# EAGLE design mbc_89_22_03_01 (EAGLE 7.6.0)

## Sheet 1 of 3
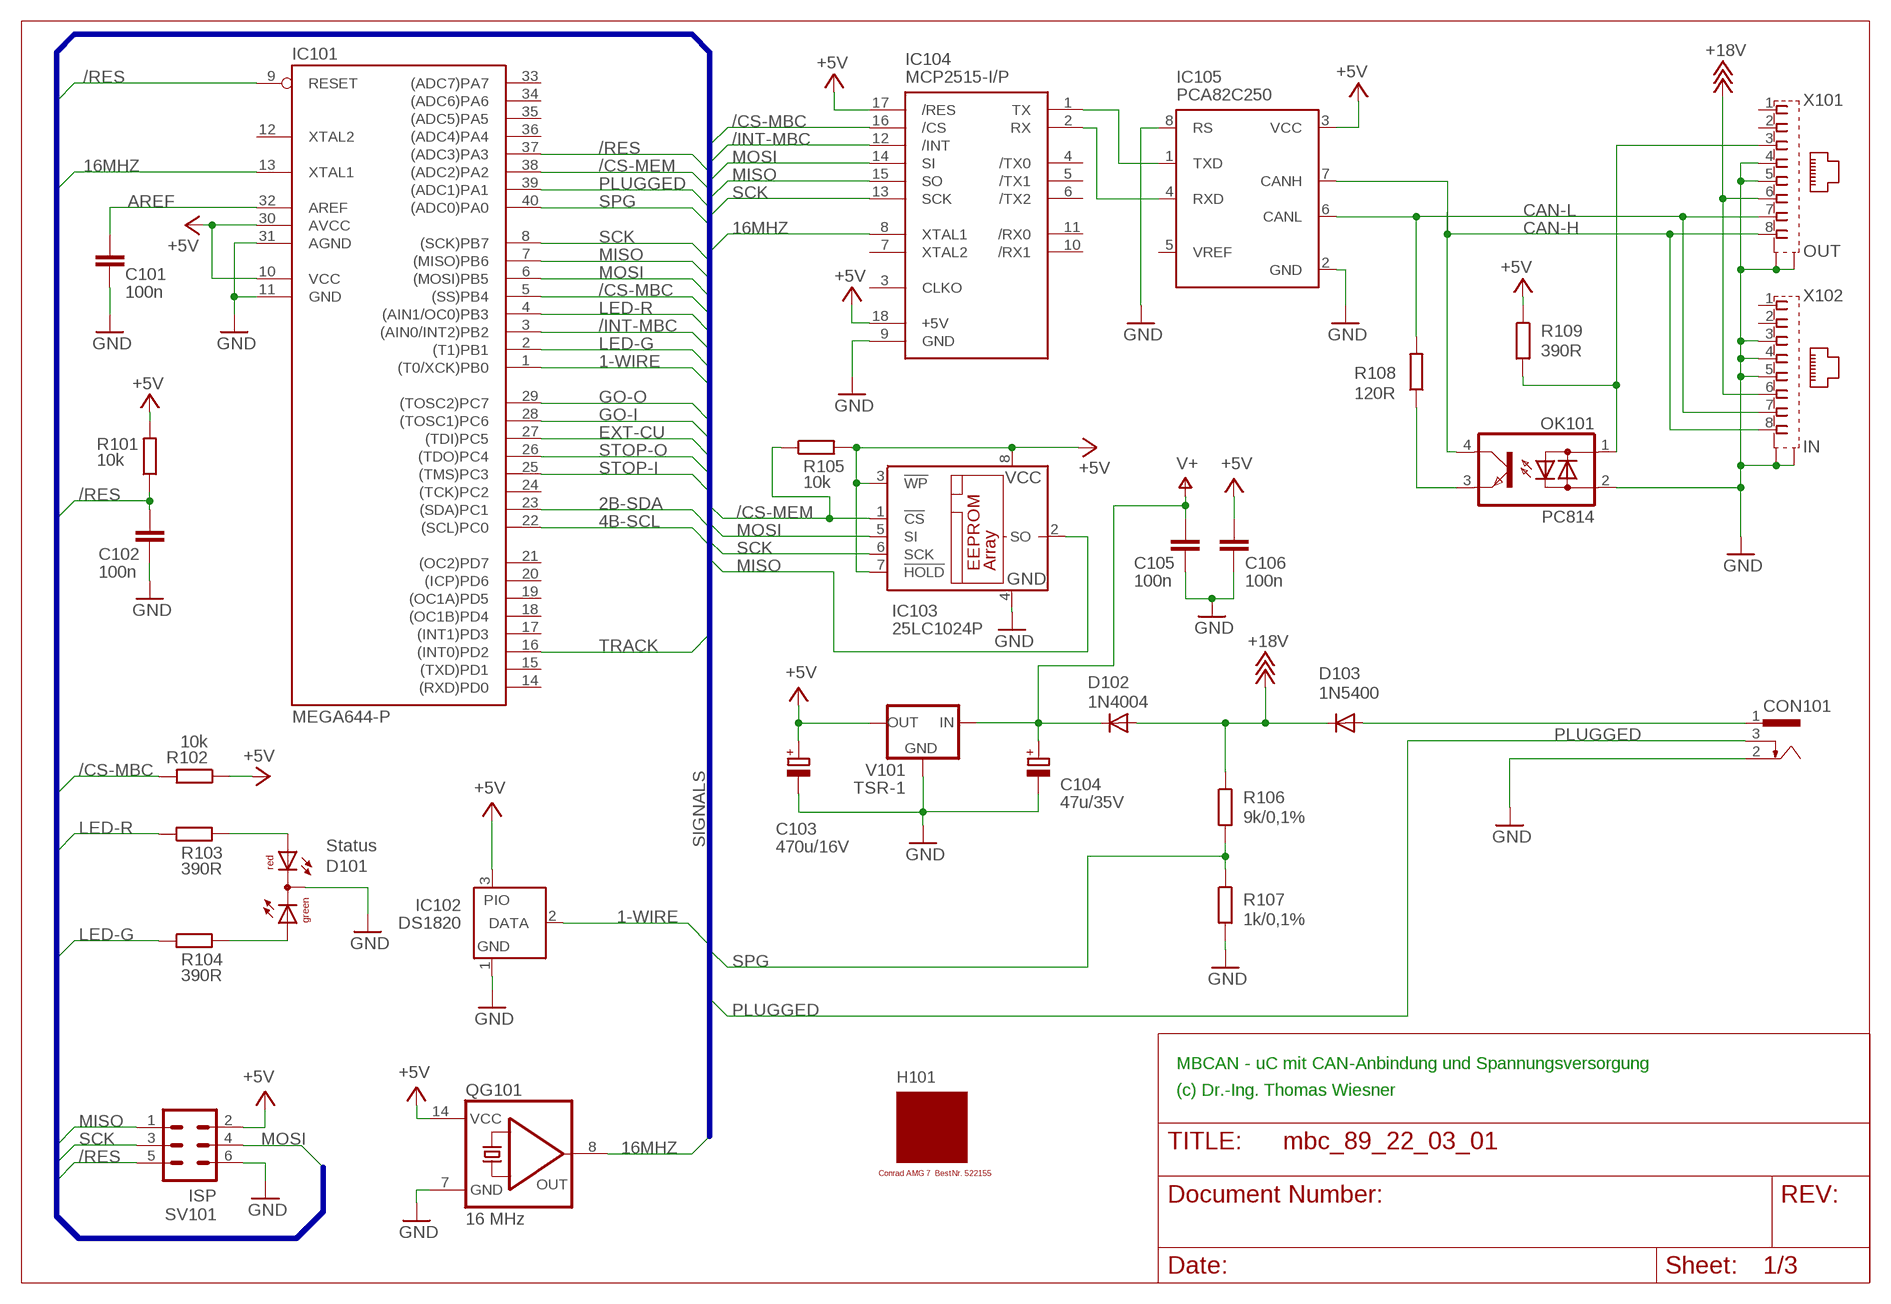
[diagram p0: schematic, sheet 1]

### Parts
C101  100n  C-EU025-025X050  [C025-025X050]
C102  100n  C-EU025-025X050  [C025-025X050]
C103  470u/16V  CPOL-EUE3.5-8  [E3,5-8]
C104  47u/35V  CPOL-EUE2.5-7  [E2,5-7]
C105  100n  C-EU025-025X050  [C025-025X050]
C106  100n  C-EU025-025X050  [C025-025X050]
CON101  POWER-JACK  [POWER-JACK]
D101  Status  DUOLED5MM  [DUOLED5MM]
D102  1N4004  [DO41-10]
D103  1N5400  [DO201-15]
H101  MODULGEHÄUSE-AMG-7  [MODULGEHÄUSE-1]
IC101  MEGA644-P  MEGA323-P  [DIL40]
IC102  DS1820  DS2405  [TO92-]
IC103  25LC1024P  25LC040P  [DIL8]
IC104  MCP2515-I/P  MCP2510-I/P  [DIL18]
IC105  PCA82C250  [DIL08]
OK101  PC814  [DIL04]
QG101  16 MHz  QG5860  [DIL14S]
R101  10k  R-EU_0207/10  [0207/10]
R102  10k  R-EU_0207/10  [0207/10]
R103  390R  R-EU_0207/10  [0207/10]
R104  390R  R-EU_0207/10  [0207/10]
R105  10k  R-EU_0207/10  [0207/10]
R106  9k/0,1%  R-EU_0207/10  [0207/10]
R107  1k/0,1%  R-EU_0207/10  [0207/10]
R108  120R  R-EU_0207/10  [0207/10]
R109  390R  R-EU_0207/10  [0207/10]
SV101  ISP  ML6  [ML6]
V101  TSR-1  [TRACO-TSR-1]
X101  OUT  0446200002  [0446200002]
X102  IN  0446200002  [0446200002]

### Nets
1-WIRE: IC101.1((T0/XCK)PB0) IC102.2(DATA)
2B-SDA: IC101.23((SDA)PC1) ; also sheet 2
4B-SCL: IC101.22((SCL)PC0) ; also sheet 2
16MHZ: IC101.13(XTAL1) IC104.8(XTAL1) QG101.8(OUT)
+5V: C103.+ C106.1 IC101.10(VCC) IC101.30(AVCC) IC102.3(PIO) IC103.3(!WP) IC103.7(!HOLD) IC103.8(VCC) IC104.17(/RES) IC104.18(+5V) IC105.3(VCC) QG101.14(VCC) R101.2 R102.1 R105.2 R109.1 SV101.2 V101.OUT ; also sheet 2
+18V: D102.A D103.C R106.1 X101.6 X102.6
/CS-MBC: IC101.5((SS)PB4) IC104.16(/CS) R102.2
/CS-MEM: IC101.38((ADC2)PA2) IC103.1(!CS) R105.1
/INT-MBC: IC101.3((AIN0/INT2)PB2) IC104.12(/INT)
/RES: C102.1 IC101.9(RESET) IC101.37((ADC3)PA3) R101.1 SV101.5
AREF: C101.1 IC101.32(AREF)
CAN-H: IC105.7(CANH) OK101.4(C) X101.8 X102.8
CAN-L: IC105.6(CANL) R108.2 X101.7 X102.7
EXT-CU: IC101.27((TDI)PC5) ; also sheet 2
GND: C101.2 C102.2 C103.- C104.- C105.2 C106.2 CON101.2 D101.K(C) IC101.11(GND) IC101.31(AGND) IC102.1(GND) IC103.4(GND) IC104.9(GND) IC105.2(GND) IC105.8(RS) OK101.2(AC2) QG101.7(GND) R107.2 SV101.6 V101.GND X101.4 X101.5 X101.S@1(S1) X101.S@2(S2) X102.3 X102.4 X102.5 X102.S@1(S1) X102.S@2(S2) ; also sheet 2
GO-I: IC101.28((TOSC1)PC6) ; also sheet 2
GO-O: IC101.29((TOSC2)PC7) ; also sheet 2
LED-G: IC101.2((T1)PB1) R104.1
LED-R: IC101.4((AIN1/OC0)PB3) R103.1
MISO: IC101.7((MISO)PB6) IC103.2(SO) IC104.15(SO) SV101.1
MOSI: IC101.6((MOSI)PB5) IC103.5(SI) IC104.14(SI) SV101.4
N$1: IC104.1(TX) IC105.1(TXD)
N$2: IC104.2(RX) IC105.4(RXD)
N$5: OK101.3(E) R108.1
N$9: D101.AR R103.2
N$11: OK101.1(AC1) R109.2 X101.3
N$13: D101.AG R104.2
PLUGGED: CON101.3 IC101.39((ADC1)PA1)
SCK: IC101.8((SCK)PB7) IC103.6(SCK) IC104.13(SCK) SV101.3
SPG: IC101.40((ADC0)PA0) R106.2 R107.1
STOP-I: IC101.25((TMS)PC3) ; also sheet 2
STOP-O: IC101.26((TDO)PC4) ; also sheet 2
TRACK: IC101.16((INT0)PD2) ; also sheet 2
V+: C104.+ C105.1 D102.C V101.IN ; also sheet 2
V-NETZTEIL: CON101.1 D103.A
Unconnected: IC101.12(XTAL2) IC101.14((RXD)PD0) IC101.15((TXD)PD1) IC101.17((INT1)PD3) IC101.18((OC1B)PD4) IC101.19((OC1A)PD5) IC101.20((ICP)PD6) IC101.21((OC2)PD7) IC101.24((TCK)PC2) IC101.33((ADC7)PA7) IC101.34((ADC6)PA6) IC101.35((ADC5)PA5) IC101.36((ADC4)PA4) IC104.3(CLKO) IC104.4(/TX0) IC104.5(/TX1) IC104.6(/TX2) IC104.7(XTAL2) IC104.10(/RX1) IC104.11(/RX0) IC105.5(VREF) X101.1 X101.2 X102.1 X102.2

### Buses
SIGNALS

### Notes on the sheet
- MBCAN - uC mit CAN-Anbindung und Spannungsversorgung
- (c) Dr.-Ing. Thomas Wiesner

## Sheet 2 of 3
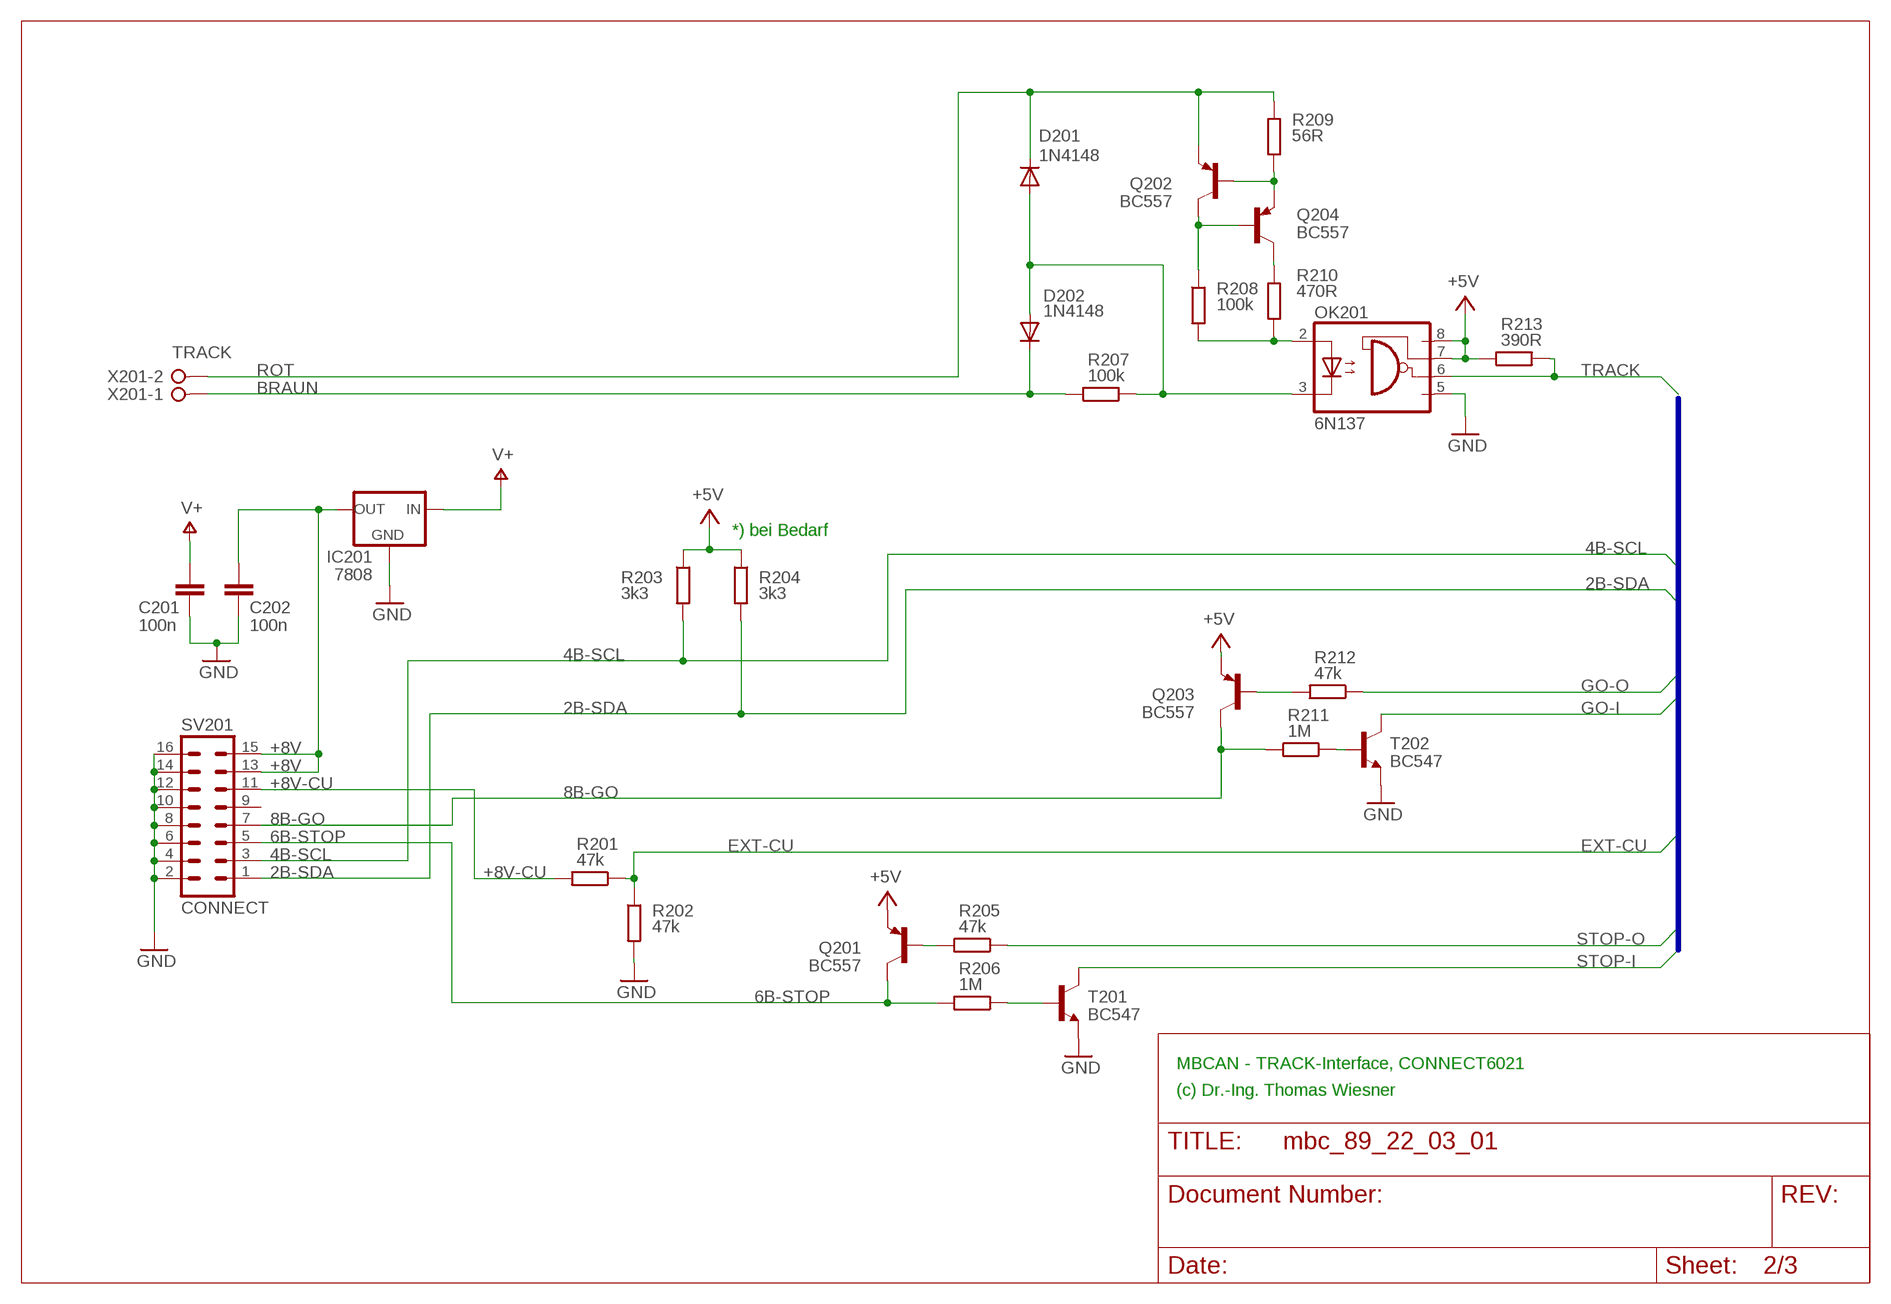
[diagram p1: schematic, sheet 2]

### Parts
C201  100n  C-EU025-025X050  [C025-025X050]
C202  100n  C-EU025-025X050  [C025-025X050]
D201  1N4148  1N4148DO35-10  [DO35-10]
D202  1N4148  1N4148DO35-10  [DO35-10]
IC201  7808  78XXL  [78XXL]
OK201  6N137  [DIL08]
Q201  BC557  [TO92]
Q202  BC557  [TO92]
Q203  BC557  [TO92]
Q204  BC557  [TO92]
R201  47k  R-EU_0207/10  [0207/10]
R202  47k  R-EU_0207/10  [0207/10]
R203  3k3  R-EU_0207/10  [0207/10]
R204  3k3  R-EU_0207/10  [0207/10]
R205  47k  R-EU_0207/10  [0207/10]
R206  1M  R-EU_0207/10  [0207/10]
R207  100k  R-EU_0207/10  [0207/10]
R208  100k  R-EU_0207/10  [0207/10]
R209  56R  R-EU_0207/10  [0207/10]
R210  470R  R-EU_0207/10  [0207/10]
R211  1M  R-EU_0207/10  [0207/10]
R212  47k  R-EU_0207/10  [0207/10]
R213  390R  R-EU_0207/10  [0207/10]
SV201  CONNECT  ML16  [ML16]
T201  BC547  [TO92]
T202  BC547  [TO92]
X201  TRACK  W237-02P  [W237-132]

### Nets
2B-SDA: R204.2 SV201.1 ; also sheet 1
4B-SCL: R203.2 SV201.3 ; also sheet 1
6B-STOP: Q201.3(C) R206.2 SV201.5
8B-GO: Q203.3(C) R211.2 SV201.7
+5V: OK201.7(VE) OK201.8(VCC) Q201.1(E) Q203.1(E) R203.1 R204.1 R213.1 ; also sheet 1
+8V: C202.1 IC201.OUT SV201.13 SV201.15
+8V-CU: R201.2 SV201.11
BRAUN: D202.C R207.2 X201.1
EXT-CU: R201.1 R202.1 ; also sheet 1
GND: C201.2 C202.2 IC201.GND OK201.5(GND) R202.2 SV201.2 SV201.4 SV201.6 SV201.8 SV201.10 SV201.12 SV201.14 SV201.16 T201.1(E) T202.1(E) ; also sheet 1
GO-I: T202.3(C) ; also sheet 1
GO-O: R212.1 ; also sheet 1
N$3: R206.1 T201.2(B)
N$4: Q201.2(B) R205.2
N$7: R211.1 T202.2(B)
N$12: Q203.2(B) R212.2
N$43: D201.A D202.A OK201.3(C) R207.1
N$53: Q202.2(B) Q204.1(E) R209.2
N$54: Q202.3(C) Q204.2(B) R208.1
N$56: Q204.3(C) R210.1
N$57: OK201.2(A) R208.2 R210.2
ROT: D201.C Q202.1(E) R209.1 X201.2
STOP-I: T201.3(C) ; also sheet 1
STOP-O: R205.1 ; also sheet 1
TRACK: OK201.6(VO) R213.2 ; also sheet 1
V+: C201.1 IC201.IN ; also sheet 1
Unconnected: SV201.9

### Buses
B$1
SIGNALS

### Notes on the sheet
- *) bei Bedarf
- MBCAN - TRACK-Interface, CONNECT6021
- (c) Dr.-Ing. Thomas Wiesner

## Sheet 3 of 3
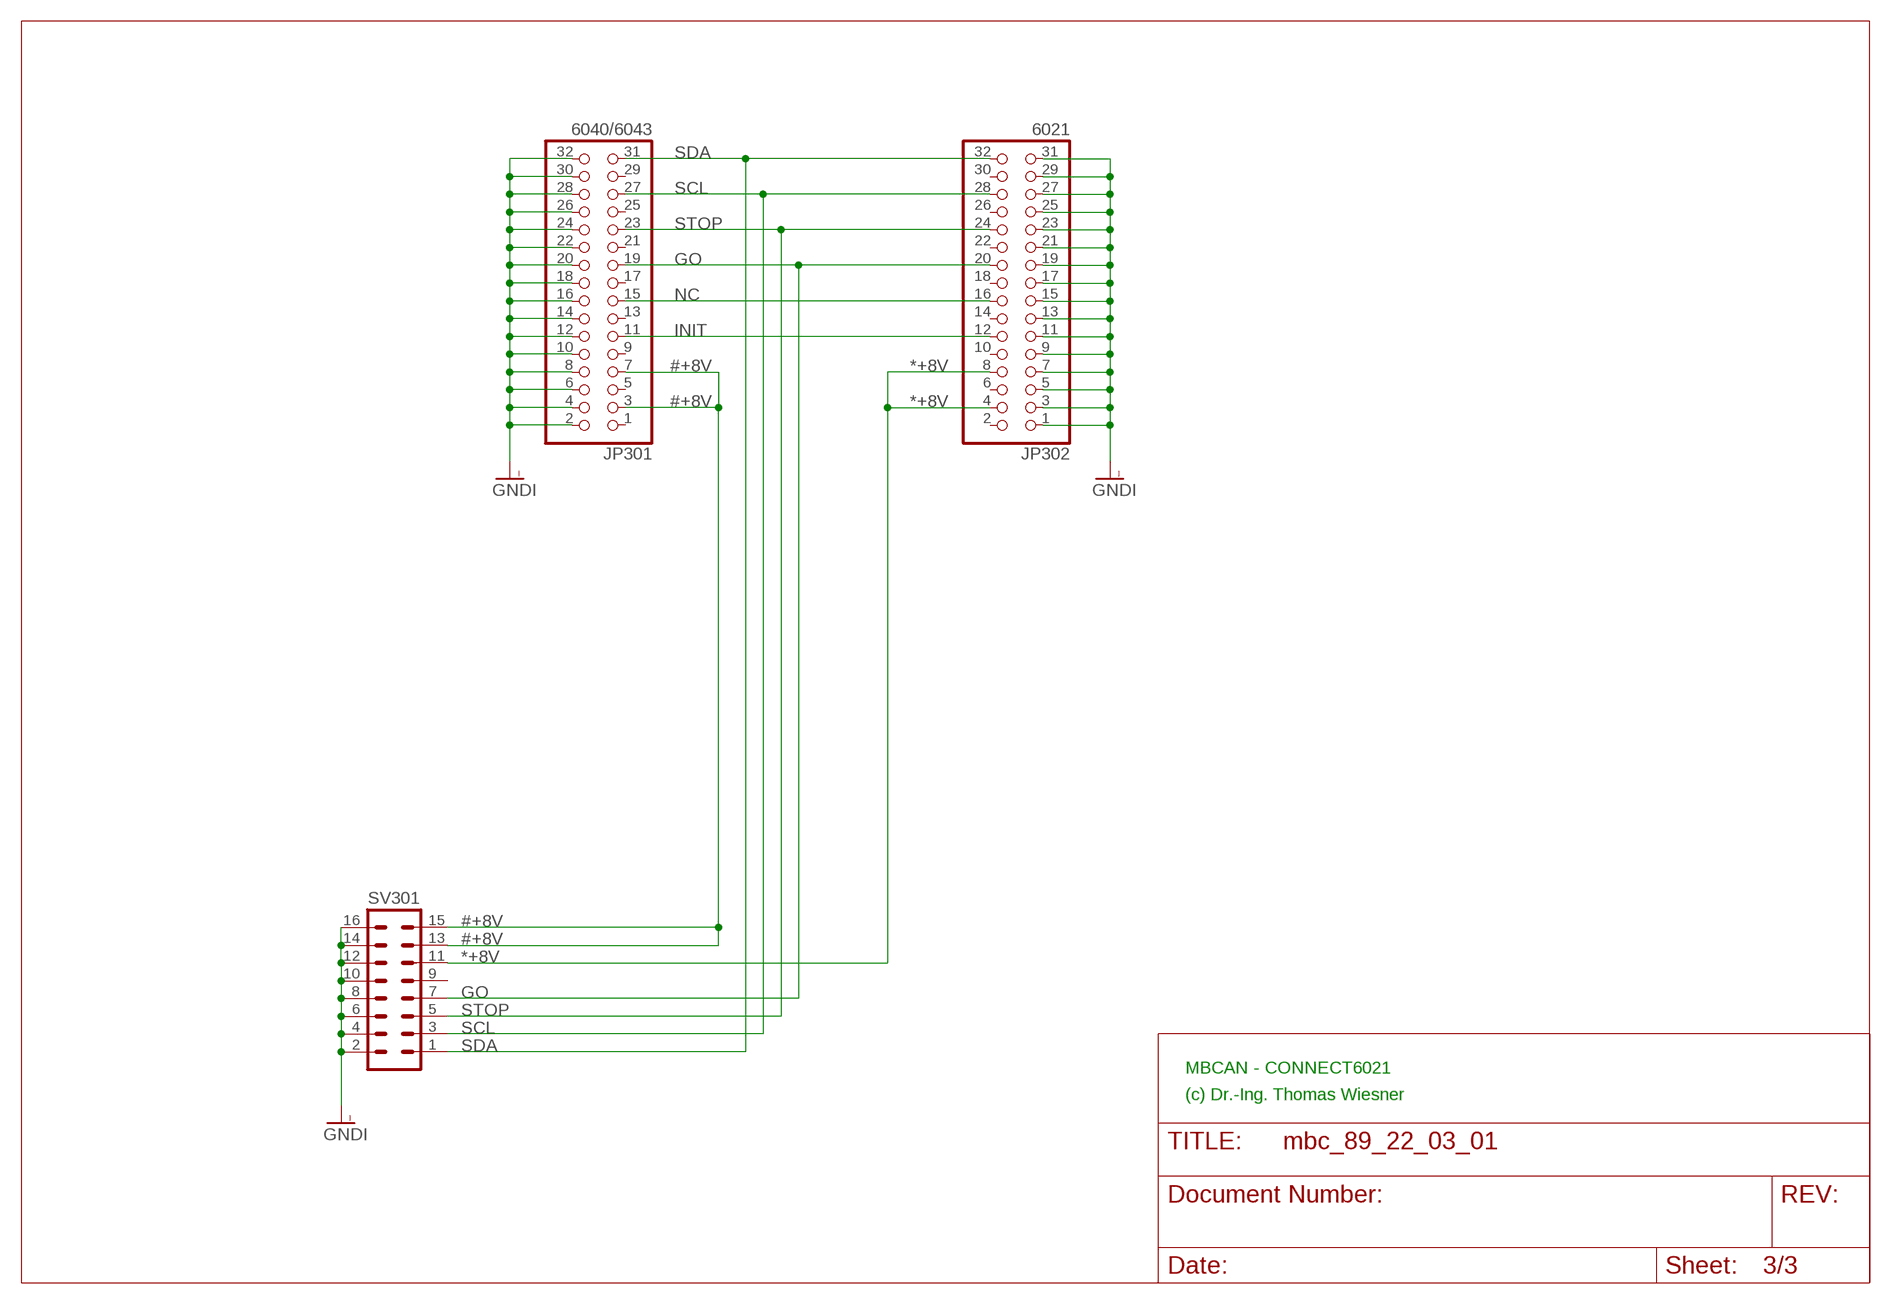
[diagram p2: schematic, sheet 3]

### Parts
JP301  6040/6043  PINHD-2X16  [2X16]
JP302  6021  PINHD-2X16  [2X16]
SV301  ML16  [ML16]

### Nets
#+8V: JP301.3 JP301.7 SV301.13 SV301.15
*+8V: JP302.4 JP302.8 SV301.11
GNDI: JP301.2 JP301.4 JP301.6 JP301.8 JP301.10 JP301.12 JP301.14 JP301.16 JP301.18 JP301.20 JP301.22 JP301.24 JP301.26 JP301.28 JP301.30 JP301.32 JP302.1 JP302.3 JP302.5 JP302.7 JP302.9 JP302.11 JP302.13 JP302.15 JP302.17 JP302.19 JP302.21 JP302.23 JP302.25 JP302.27 JP302.29 JP302.31 SV301.2 SV301.4 SV301.6 SV301.8 SV301.10 SV301.12 SV301.14 SV301.16
GO: JP301.19 JP302.20 SV301.7
INIT: JP301.11 JP302.12
NC: JP301.15 JP302.16
SCL: JP301.27 JP302.28 SV301.3
SDA: JP301.31 JP302.32 SV301.1
STOP: JP301.23 JP302.24 SV301.5
Unconnected: JP301.1 JP301.5 JP301.9 JP301.13 JP301.17 JP301.21 JP301.25 JP301.29 JP302.2 JP302.6 JP302.10 JP302.14 JP302.18 JP302.22 JP302.26 JP302.30 SV301.9

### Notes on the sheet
- MBCAN - CONNECT6021
- (c) Dr.-Ing. Thomas Wiesner

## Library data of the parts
C101 C102 C105 C106 C201 C202 = rcl:C-EU: CAPACITOR, European symbol
C103 C104 = rcl:CPOL-EU: POLARIZED CAPACITOR, European symbol
CON101 = mbc:POWER-JACK
D101 = led:DUOLED5MM: DUO LED 2 colors, 5 mm, round
D102 = diode:1N4004: DIODE
D103 = diode:1N5400: DIODE
D201 D202 = diode:1N4148: DIODE
H101 = mbc:MODULGEHÄUSE-AMG-7: Gehäuse
IC101 = atmel:MEGA323-P: MICROCONTROLLER 32 Kbytes FLASH 2 Kbytes SRAM 1 Kbytes EEPROM USART 8-channel 10 bit ADC Source: avr.lbr; OC_FARNELL: unknown; OC_NEWARK: unknown
IC102 = maxim:DS2405: Addressable Switch DALLAS Semiconductor; MF: DALLAS SEMICONDUCTOR; MPN: DS2405; OC_FARNELL: 1188025; OC_NEWARK: 06F4645
IC103 = microchip:25*: Serial EEPROM 4K/ 8K , SPI bus; MF: MICROCHIP; MPN: 25LC040/P; OC_FARNELL: 9758100; OC_NEWARK: 96K4091
IC104 = mbc:MCP2510: BASIC-CAN 2.0a Controller Stand-alone CAN controller von Microchip
IC105 = micro-philips:PCA82C250: CAN CONTROLLER INTERFACE; OC_FARNELL: 3692358; OC_NEWARK: unknown
IC201 = v-reg:78XXL: VOLTAGE REGULATOR
JP301 JP302 = pinhead:PINHD-2X16: PIN HEADER
OK101 = optocoupler:PC814: SHARP OPTO COUPLER; OC_FARNELL: 9707662; OC_NEWARK: unknown
OK201 = optocoupler:6N137: MOTOROLA OPTO COUPLER; MPN: 6N137; OC_FARNELL: 1328376; OC_NEWARK: 52M1895
Q201-Q204 = transistor-pnp:BC557: PNP Transistor
QG101 = crystal:QG5860: CRYSTAL RESONATOR; OC_FARNELL: unknown; OC_NEWARK: unknown
R101-R109 R201-R213 = resistor:R-EU_: RESISTOR, European symbol
SV101 = con-ml:ML6: HARTING; OC_FARNELL: unknown; OC_NEWARK: unknown
SV201 SV301 = con-ml:ML16: HARTING; OC_FARNELL: unknown; OC_NEWARK: unknown
T201 T202 = transistor:BC547: NPN TRANSISTOR
V101 = mbc:TSR-1: Spannungsregler Hersteller: TRACO Typ: TSR-1 5V: TSR 1-2450 Spg: 5V Strom: 1A Reichelt TSR 1-2450
X101 X102 = mbc:0446200002: RJ-45 INVERTED MODULAR JACK ASSEMBLY WITH RJ-11 KEEPOUT FEATURE Source: Data sheet MOLEX 0446200002 BUCHSE, RJ45, GESCHIRMT Source: Farnell; MF: MOLEX; MPN: 0446200002; OC_FARNELL: 9251910
X201 = con-wago-508:W237-02P: WAGO SREW CLAMP; OC_FARNELL: unknown; OC_NEWARK: unknown

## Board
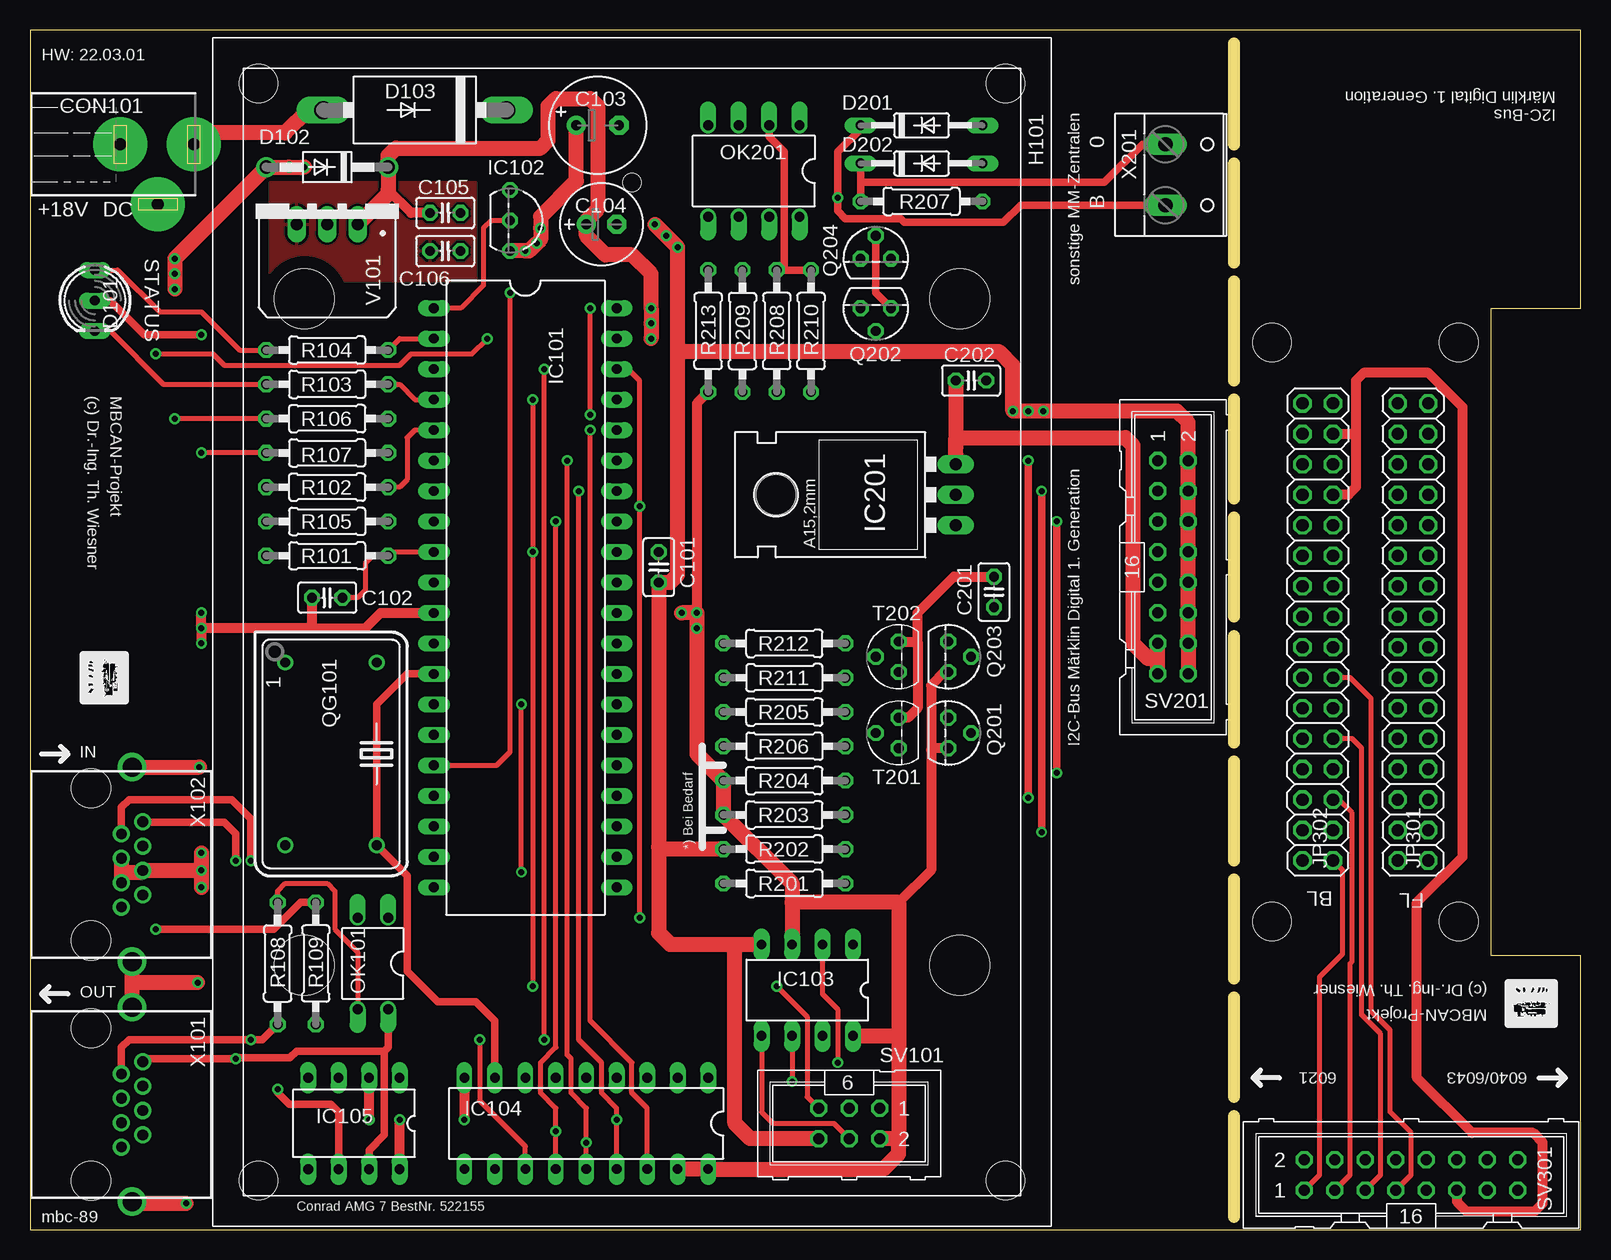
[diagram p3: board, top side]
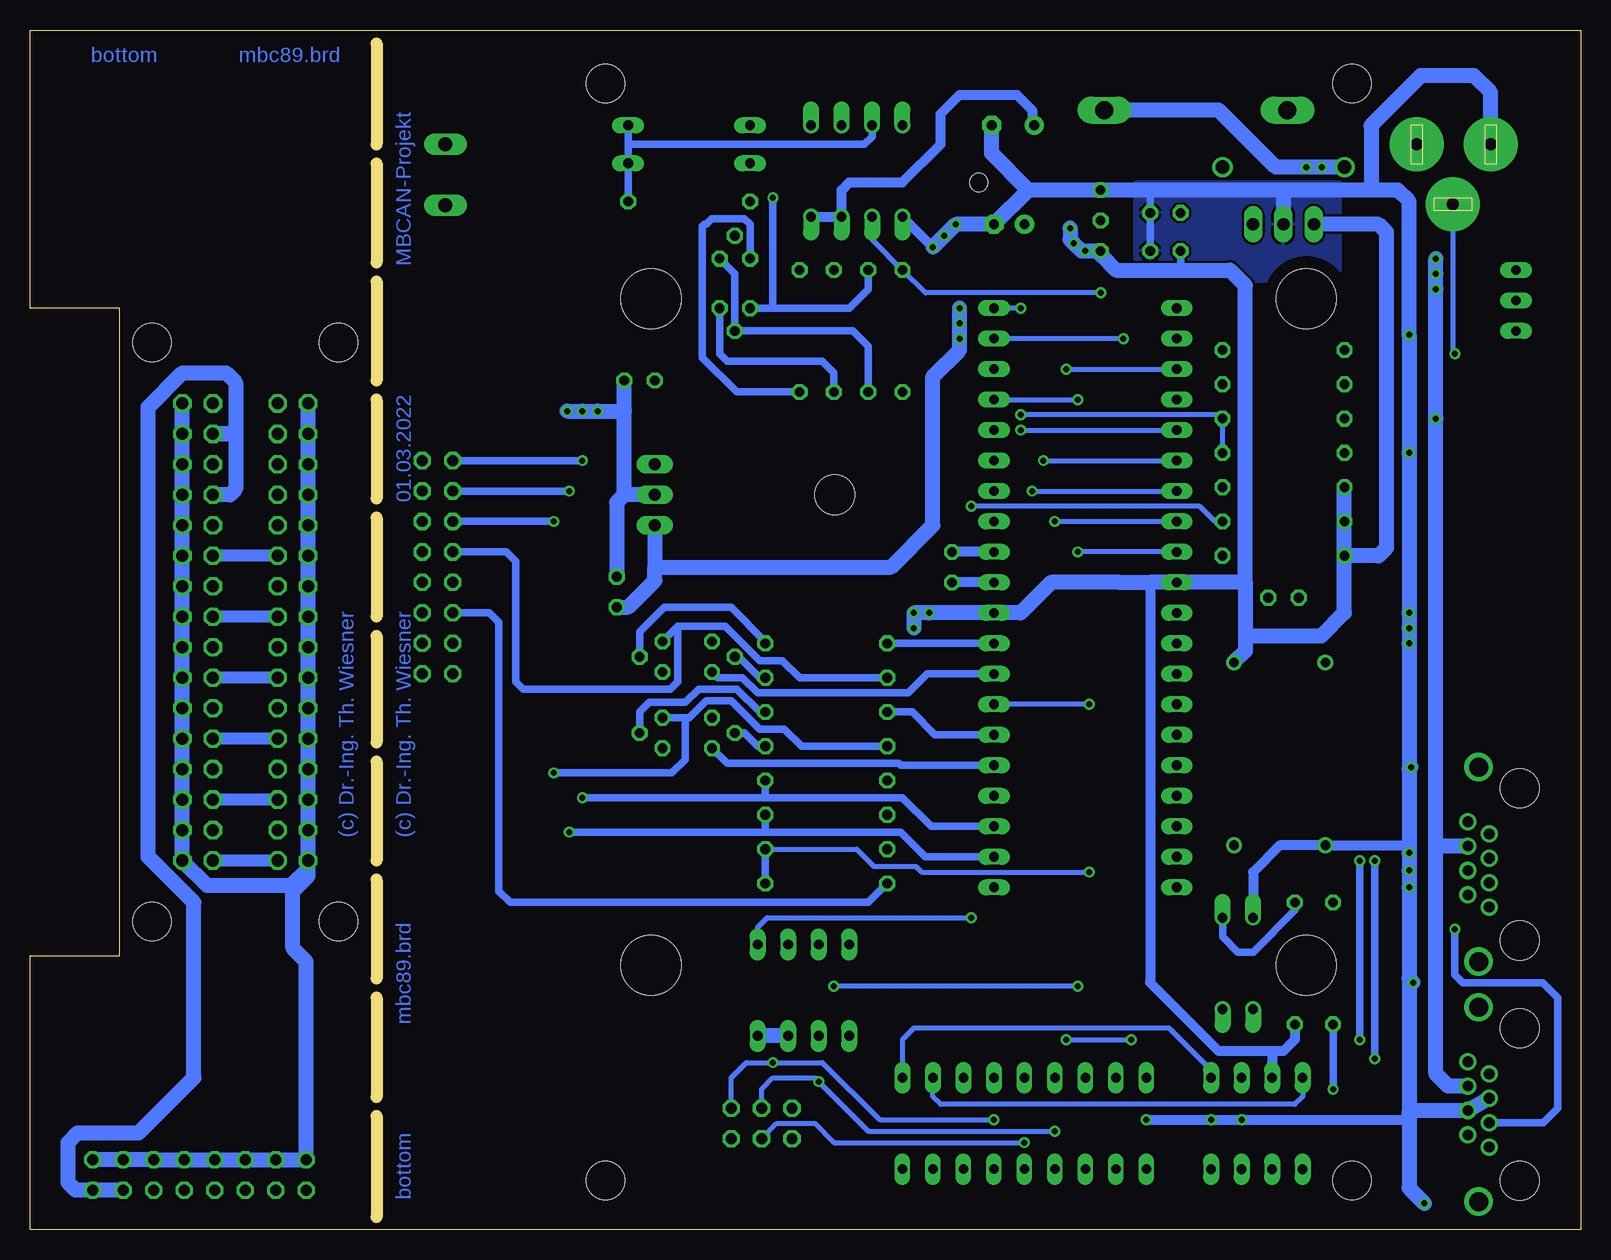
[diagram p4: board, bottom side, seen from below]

Size 129.22 x 99.99 mm. Coordinates in mm from the lower left corner, seen from the top.
Outline: 0,99.99 0,0 129.21,0 129.22,22.84 121.76,22.84 121.76,76.81 129.21,76.81 129.21,99.99 0,99.99
Copper layers (1*16): Top 0.035mm / dielectric 1.5mm / Bottom 0.035mm
Design rules "default *": minimum track width 10mil, minimum drill 0.5mm, track to track 8mil, track to pad 8mil, pad to pad 8mil, via to via 8mil, smd to smd 8mil, copper to edge 40mil, drill to drill 8mil, minimum pad ring 10mil, minimum via ring 8mil, stop-mask expansion 4mil, vias tented up to drill 0mil, thermal gap 10mil
Holes 3.2 mm at 103.5,25.7 103.5,73.96 119.06,73.96 119.06,25.7
Milling: 10 lines

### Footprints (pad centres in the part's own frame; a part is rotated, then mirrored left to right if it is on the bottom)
C025-025X050 = drill 0.813 octagon: 1 -1.27,0; 2 1.27,0
E3,5-8 = drill 0.813 pad 1.6: + -1.778,0 | drill 0.813 pad 1.6 octagon: - 1.778,0
E2,5-7 = drill 0.813 pad 1.6: + -1.27,0 | drill 0.813 pad 1.6 octagon: - 1.27,0
POWER-JACK = drill 1 pad 4.5: 1 0,6.03; 2 0,-0.12; 3 5,3.03
DUOLED5MM = drill 0.813 long: AG -2.54,0; AR 2.54,0; K 0,0
DO41-10 = drill 1.118: A 5.08,0; C -5.08,0
DO201-15 = drill 1.499 long: A 7.62,0; C -7.62,0
DO35-10 = drill 0.813 long: A 5.08,0; C -5.08,0
MODULGEHÄUSE-1 = hole 3.2: -45.72,-31.115; -45.72,31.115; 45.72,31.115; 45.72,-31.115 | hole 5: -27.781,-27.305; 27.781,-27.305; -27.781,27.305; 27.781,27.305 | hole 1.5: -37.465,0
DIL40 = drill 0.813 long: 1 -24.13,-7.62; 2 -21.59,-7.62; 3 -19.05,-7.62; 4 -16.51,-7.62; 5 -13.97,-7.62; 6 -11.43,-7.62; 7 -8.89,-7.62; 8 -6.35,-7.62; 9 -3.81,-7.62; 10 -1.27,-7.62; 11 1.27,-7.62; 12 3.81,-7.62; 13 6.35,-7.62; 14 8.89,-7.62; 15 11.43,-7.62; 16 13.97,-7.62; 17 16.51,-7.62; 18 19.05,-7.62; 19 21.59,-7.62; 20 24.13,-7.62; 21 24.13,7.62; 22 21.59,7.62; 23 19.05,7.62; 24 16.51,7.62; 25 13.97,7.62; 26 11.43,7.62; 27 8.89,7.62; 28 6.35,7.62; 29 3.81,7.62; 30 1.27,7.62; 31 -1.27,7.62; 32 -3.81,7.62; 33 -6.35,7.62; 34 -8.89,7.62; 35 -11.43,7.62; 36 -13.97,7.62; 37 -16.51,7.62; 38 -19.05,7.62; 39 -21.59,7.62; 40 -24.13,7.62
TO92- = drill 0.813 octagon: 1 -2.54,0; 2 0,0; 3 2.54,0
DIL8 = drill 0.813 long: 1 -3.81,-3.81; 2 -1.27,-3.81; 3 1.27,-3.81; 4 3.81,-3.81; 5 3.81,3.81; 6 1.27,3.81; 7 -1.27,3.81; 8 -3.81,3.81
DIL18 = drill 0.813 long: 1 -10.16,-3.81; 2 -7.62,-3.81; 3 -5.08,-3.81; 4 -2.54,-3.81 | drill 0.8 long: 5 0,-3.81; 6 2.54,-3.81; 7 5.08,-3.81; 8 7.62,-3.81; 9 10.16,-3.81; 10 10.16,3.81; 11 7.62,3.81; 12 5.08,3.81; 13 2.54,3.81; 14 0,3.81; 15 -2.54,3.81; 16 -5.08,3.81; 17 -7.62,3.81; 18 -10.16,3.81
DIL08 = drill 0.813 long: 1 -3.81,-3.81; 2 -1.27,-3.81; 3 1.27,-3.81; 4 3.81,-3.81; 5 3.81,3.81; 6 1.27,3.81; 7 -1.27,3.81; 8 -3.81,3.81
78XXL = drill 1.016 long: GND 0,-3.81; IN -2.54,-3.81; OUT 2.54,-3.81 | hole 3.302: 0,11.176
2X16 = drill 1.016 octagon: 1 -19.05,-1.27; 2 -19.05,1.27; 3 -16.51,-1.27; 4 -16.51,1.27; 5 -13.97,-1.27; 6 -13.97,1.27; 7 -11.43,-1.27; 8 -11.43,1.27; 9 -8.89,-1.27; 10 -8.89,1.27; 11 -6.35,-1.27; 12 -6.35,1.27; 13 -3.81,-1.27; 14 -3.81,1.27; 15 -1.27,-1.27; 16 -1.27,1.27; 17 1.27,-1.27; 18 1.27,1.27; 19 3.81,-1.27; 20 3.81,1.27; 21 6.35,-1.27; 22 6.35,1.27; 23 8.89,-1.27; 24 8.89,1.27; 25 11.43,-1.27; 26 11.43,1.27; 27 13.97,-1.27; 28 13.97,1.27; 29 16.51,-1.27; 30 16.51,1.27; 31 19.05,-1.27; 32 19.05,1.27
DIL04 = drill 0.813 offset: 1 -1.27,-3.81; 2 1.27,-3.81; 3 1.27,3.81; 4 -1.27,3.81
DIL08' = drill 0.813 offset: 1 -3.81,-3.81; 2 -1.27,-3.81; 3 1.27,-3.81; 4 3.81,-3.81; 5 3.81,3.81; 6 1.27,3.81; 7 -1.27,3.81; 8 -3.81,3.81
TO92 = drill 0.813 octagon: 1 1.27,0; 2 0,1.905; 3 -1.27,0
DIL14S = drill 0.813: 1 -7.62,-3.81; 7 7.62,-3.81; 8 7.62,3.81; 14 -7.62,3.81
0207/10 = drill 0.813 octagon: 1 -5.08,0; 2 5.08,0
ML6 = drill 0.914 octagon: 1 -2.54,-1.27; 2 -2.54,1.27; 3 0,-1.27; 4 0,1.27; 5 2.54,-1.27; 6 2.54,1.27
ML16 = drill 0.914 octagon: 1 -8.89,-1.27; 2 -8.89,1.27; 3 -6.35,-1.27; 4 -6.35,1.27; 5 -3.81,-1.27; 6 -3.81,1.27; 7 -1.27,-1.27; 8 -1.27,1.27; 9 1.27,-1.27; 10 1.27,1.27; 11 3.81,-1.27; 12 3.81,1.27; 13 6.35,-1.27; 14 6.35,1.27; 15 8.89,-1.27; 16 8.89,1.27
TRACO-TSR-1 = drill 1.016 long: GND 0,2.54; IN -2.54,2.54; OUT 2.54,2.54
0446200002 = drill 0.889 pad 1.422: 1 3.556,2.54; 2 2.54,4.318; 3 1.524,2.54; 4 0.508,4.318; 5 -0.508,2.54; 6 -1.524,4.318; 7 -2.54,2.54; 8 -3.556,4.318 | drill 1.575 pad 2.286: S@1 -8.103,3.429; S@2 8.103,3.429 | hole 3.251: 6.35,0; -6.35,0
W237-132 = drill 1.194 long: 1 -2.54,-0.635; 2 2.54,-0.635

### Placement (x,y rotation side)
C101  52.39,55.22 270 top
C102  24.77,52.68 180 top
C103  47.31,92.06 0 top
C104  47.62,83.8 0 top
C105  34.61,84.75 0 top
C106  34.61,81.58 0 top
C201  80.33,53.16 90 top
C202  78.42,70.78 0 top
CON101  7.62,90.47 270 top
D101  5.4,77.45 270 top
D102  24.77,88.56 180 top
D103  32.07,93.33 180 top
D201  74.3,92.06 0 top
D202  74.3,88.88 0 top
H101  50.16,49.83 270 top
IC101  41.27,52.68 270 top
IC102  40.01,84.12 270 top
IC103  64.77,19.98 180 top
IC104  46.35,8.87 180 top
IC105  26.99,8.87 180 top
IC201  73.34,61.26 90 top
JP301  115.25,49.83 270 top
JP302  107.31,49.83 270 top
OK101  28.57,22.21 180 top
OK201  6N137  [DIL08']  60.33,88.25 180 top
Q201  76.52,41.41 270 top
Q202  70.48,76.81 180 top
Q203  76.52,47.76 270 top
Q204  70.48,80.94 0 top
QG101  25.08,39.67 270 top
R101  24.77,56.18 180 top
R102  24.77,61.89 0 top
R103  24.77,70.47 180 top
R104  24.77,73.32 180 top
R105  24.77,59.03 180 top
R106  24.77,67.61 0 top
R107  24.77,64.75 180 top
R108  20.64,22.21 270 top
R109  23.81,22.21 90 top
R201  62.87,28.87 180 top
R202  62.87,31.73 180 top
R203  62.87,34.59 0 top
R204  62.87,37.45 0 top
R205  62.87,43.16 0 top
R206  62.87,40.3 180 top
R207  74.3,85.7 180 top
R208  62.23,74.91 90 top
R209  59.37,74.91 270 top
R210  65.09,74.91 90 top
R211  62.87,46.02 180 top
R212  62.87,48.88 0 top
R213  56.52,74.91 90 top
SV101  68.26,8.87 180 top
SV201  95.25,55.22 270 top
SV301  115.09,4.58 0 top
T201  72.39,41.41 90 top
T202  72.39,47.76 90 top
V101  24.77,86.34 180 top
X101  5.08,10.46 270 top
X102  5.08,30.46 270 top
X201  95.25,87.93 270 top

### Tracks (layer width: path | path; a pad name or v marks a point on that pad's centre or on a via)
1-WIRE
  Top 0.406: IC101.1 35.88,76.81 37.78,78.72 37.78,83.48 38.42,84.12 IC102.2
2B-SDA  (via drill 0.5)
  Top 0.61: v83.19,64.12 v83.19,36.02
  Bottom 0.61: SV201.1 v83.19,64.12 | v83.19,36.02 67.94,36.02 | 67.94,36.02 56.52,36.02 54.13,33.63 IC101.23 | R204.2 67.94,36.02
4B-SCL  (via drill 0.5)
  Top 0.61: v84.3,61.57 v84.3,33.16
  Bottom 0.61: SV201.3 v84.3,61.57 | v84.3,33.16 67.94,33.16 | 67.94,33.16 56.67,33.16 54.61,31.09 IC101.22 | R203.2 67.94,33.16
6B-STOP  (via drill 0.5)
  Top 0.61: v85.57,59.03 v85.57,38.08
  Bottom 0.61: R206.2 64.93,40.3 66.36,41.73 68.42,41.73 70.8,44.11 72.87,44.11 74.3,42.68 74.61,42.68 | SV201.5 v85.57,59.03 | v85.57,38.08 75.72,38.08 74.61,39.19 74.61,42.68 | 74.61,42.68 Q201.3
8B-GO
  Bottom 0.61: R211.2 65.09,46.02 66.52,47.45 68.42,47.45 71.28,50.3 75.25,50.3 | Q203.3 75.25,50.3 | 75.25,50.3 75.25,45.7 75.88,45.06 88.11,45.06 88.74,45.7 88.74,55.7 89.53,56.49 SV201.7
16MHZ
  Top 0.61: IC104.8 38.73,17.44 37.15,19.03 33.97,19.03 31.43,21.57 31.43,29.51 QG101.8 28.89,43.79 31.43,46.33 IC101.13
#+8V
  Bottom 0.813: SV301.15 SV301.13
  Bottom 1.27: SV301.13 125.41,3.31 126.05,3.95 126.05,7.28 125.25,8.08 120.17,8.08 115.57,12.68 115.57,27.29 119.38,31.09 119.38,68.56 116.52,71.42 112.87,71.42 112.08,70.62 112.08,66.5 | 112.08,66.5 112.08,66.34 | 112.08,66.34 JP301.3 112.24,66.34 112.08,66.5 | 112.08,66.34 112.08,61.73 112.55,61.26 JP301.7
*+8V
  Top 0.61: 110.49,66.34 110.01,66.34
  Top 0.813: JP302.4 110.01,66.34 | JP302.8 109.86,61.26 110.49,61.89 110.49,66.34 110.49,70.78 111.12,71.42 116.52,71.42 119.38,68.56 119.38,31.09 115.57,27.29 115.57,12.68 120.17,8.08 125.25,8.08 126.05,7.28 126.05,2.2 125.41,1.57 119.7,1.57 118.9,2.36 SV301.11
+5V  (via drill 0.5)
  Top 0.813: R213.1 55.56,68.88 v55.56,51.41 | Q203.1 76.2,46.49 75.09,45.38 75.09,39.98 | 75.09,39.98 75.09,29.98 72.39,27.29 | Q201.1 75.41,40.14 75.09,39.98
  Top 1.27: C103.+ 45.53,87.42 42.55,84.44 v42.55,83.48 42.55,82.53 v42.23,82.21 41.59,81.58 v41.27,81.58 IC102.3 | IC104.17 IC104.18 71.12,5.06 72.39,6.33 72.39,7.6 | IC103.8 72.39,16.17 | 72.39,16.17 72.39,7.6 | 72.39,7.6 SV101.2 | 72.39,16.17 72.39,27.29 63.5,27.29 | 63.5,27.29 IC103.3 | v54.29,51.41 v55.56,51.41 v55.56,50.14 55.56,39.67 R204.1 R203.1 63.5,28.87 63.5,27.29
  Bottom 0.406: 15.88,69.51 16.19,56.81
  Bottom 0.61: C106.1 33.34,79.99
  Bottom 0.813: 27.62,49.51 26.67,49.51 | 35.88,53.95 35.88,20.62 30.16,14.9 25.72,14.9 | R109.1 23.81,15.86 24.77,14.9 25.72,14.9 | 25.72,14.9 IC105.3 25.72,13.95 | OK201.8 OK201.7 61.59,86.66 60.96,87.29 56.52,87.29 53.34,90.47 53.34,93.01 51.75,94.59 46.99,94.59 45.72,93.33 45.72,92.25 C103.+
  Bottom 1.27: 27.94,53.95 IC101.10 35.88,53.95 37.15,53.95 38.42,53.95 44.13,53.95 46.67,51.41 IC101.30 v54.29,51.41 v55.56,51.41 v55.56,50.14 | R101.2 19.68,51.41 21.59,49.51 26.67,49.51 27.94,49.51 | 27.94,53.95 27.94,78.72 29.21,79.99 33.34,79.99 38.73,79.99 40.01,81.26 IC102.3 41.59,81.58 v42.23,82.21 42.55,82.53 v42.55,83.48 | 27.94,53.95 27.94,49.51 | V101.OUT 16.83,83.8 16.19,83.17 16.19,56.81 16.83,56.18 R101.2 | IC103.7 IC103.8 | R101.2 R105.2 R102.1 | 27.94,49.51 27.94,48.24 QG101.14
  pour Top: 37.15,87.29 37.15,79.04 20,79.04 20,87.29
+8V
  Top 0.813: 93.98,47.6 SV201.15
  Top 1.016: 93.19,47.6 93.98,47.6
  Top 1.27: C202.1 77.15,66.02 | IC201.OUT 77.15,64.59 77.15,65.23 77.15,66.02 | 77.15,66.02 91.28,66.02 91.92,65.39 91.92,48.88 93.19,47.6 | SV201.15 SV201.13
+8V-CU
  Bottom 0.61: R201.2 59.37,27.29 89.22,27.29 90.17,28.24 90.17,50.62 90.96,51.41 SV201.11
+18V  (via drill 0.5)
  Top 0.406: R106.1 v12.06,67.61
  Top 1.27: v12.06,78.4 v12.06,79.67 v12.06,80.94 D102.A v21.59,88.56 v22.86,88.56
  Bottom 1.27: D103.C 30.16,93.33 25.4,88.56 v22.86,88.56 v21.59,88.56 D102.A | X101.6 11.05,11.98 12.06,13 12.06,32.05 | 12.06,32.05 v12.06,67.61 v12.06,78.4 v12.06,79.67 v12.06,80.94 | X102.6 12,31.98 12.06,32.05
/CS-MBC  (via drill 0.5)
  Top 0.406: IC104.16 51.44,10.14 50.16,11.41 50.16,13.95 46.67,17.44 v46.67,66.66 | IC101.5 32.07,66.66 31.43,66.02 31.43,62.53 30.8,61.89 R102.2
  Bottom 0.406: v46.67,66.66 IC101.5
/CS-MEM  (via drill 0.5)
  Top 0.406: v50.8,26.02 v50.8,60.3 50.8,70.78 49.85,71.73 IC101.38
  Bottom 0.406: IC103.1 68.58,25.22 67.79,26.02 v50.8,26.02 | R105.1 30.48,59.03 31.75,60.3 v50.8,60.3
/INT-MBC  (via drill 0.5)
  Top 0.406: IC104.12 41.27,6.97 37.47,10.78 v37.47,15.86 | v42.86,15.86 v42.86,71.73
  Bottom 0.406: v42.86,71.73 IC101.3 | v42.86,15.86 v37.47,15.86
/RES  (via drill 0.5)
  Top 0.406: IC101.9 30.16,56.49 R101.1 28.57,56.18 27.94,55.54 27.94,53.32 27.3,52.68 C102.1 | v41.91,20.3 v41.91,56.49 v41.91,69.2 | v62.23,20.3 64.77,17.76 64.77,11.09 SV101.5
  Bottom 0.406: IC101.9 v41.91,56.49 | v41.91,20.3 v62.23,20.3 | IC101.37 v41.91,69.2
AREF
  Bottom 0.813: IC101.32 C101.1
BRAUN
  Top 0.61: R207.2 D202.C 69.22,87.29 89.53,87.29 92.71,90.47 X201.1
CAN-H  (via drill 0.5)
  Top 0.61: OK101.4 29.84,15.22 29.53,14.9 | 29.53,14.9 29.53,7.92 28.26,6.65 IC105.7 | 29.53,14.9 22.23,14.9 21.65,14.33 17.14,14.33 v17.14,14.27 9.4,14.27 X101.8 | X102.8 9.4,33.95 16.19,33.95 17.14,33 v17.14,30.78
  Bottom 0.61: v17.14,30.78 v17.14,14.27
CAN-L  (via drill 0.5)
  Top 0.61: IC105.6 25.72,9.82 25.08,10.46 21.59,10.46 20.64,11.41 v20.64,11.73 | R108.2 19.37,15.86 v18.41,15.86 8.26,15.86 7.62,15.22 X101.7 | v18.41,30.78 18.41,34.27 16.83,35.86 8.26,35.86 7.62,35.22 X102.7
  Bottom 0.61: v20.64,11.73 R108.2 | v18.41,30.78 v18.41,15.86
EXT-CU  (via drill 0.5)
  Top 0.406: v40.96,29.82 v40.96,43.79
  Bottom 0.406: R202.1 60.33,31.73 58.9,30.3 55.4,30.3 54.93,29.82 v40.96,29.82 | v40.96,43.79 IC101.27
  Bottom 0.61: R201.1 R202.1
GND  (via drill 0.5)
  Top 0.406: R107.2 v14.29,64.75
  Top 0.61: D101.K 6.67,77.45 9.53,74.59 v14.29,74.59
  Top 0.813: 23.5,50.14 27.94,50.14 29.21,51.41 IC101.11 | C102.2 23.5,50.14 | IC105.8 v30.8,9.19 | v28.26,9.19 IC105.2 | IC104.9 v36.2,9.19 | 23.5,50.14 v14.29,50.14 | v14.29,50.14 v14.29,51.41 | v14.29,50.14 v14.29,48.88 | SV201.10 SV201.8 | 73.98,49.03 73.98,43.48 73.18,42.68 T201.1 | T202.1 73.98,49.03 | 73.98,49.03 73.98,51.41 76.99,54.43 C201.2
  Top 1.27: SV101.6 60.01,7.6 58.74,8.87 58.74,23.79 | 58.74,23.79 IC103.4 | 58.74,23.79 53.34,23.79 52.39,24.75 52.39,31.89 | 52.39,31.89 C101.2 53.34,53.95 53.98,54.59 53.98,73.16 | 53.98,73.16 v53.98,81.9 v53.02,82.85 v52.07,83.8 | 7.62,29.82 X102.3 | X102.5 7.62,29.82 | 7.62,29.82 9.4,29.82 X102.4 v14.29,29.95 | X101.S@2 8.51,2.2 v13.02,2.2 | X101.S@1 8.51,20.62 | 8.51,20.62 X102.S@2 | v13.97,20.62 8.51,20.62 | X102.S@1 v14.12,38.56 | v14.29,31.41 v14.29,28.55 | SV201.8 SV201.6 SV201.4 SV201.2 | 53.98,73.16 80.8,73.16 81.92,72.05 v81.92,68.24 v83.19,68.24 v84.45,68.24 95.57,68.24 96.52,67.29 SV201.10 SV201.12 SV201.14 SV201.16 | R202.2 52.55,31.73 52.39,31.89
  Bottom 0.61: 36.2,86.66 35.88,86.66 C105.2 C106.2
  Bottom 0.813: IC101.31 C101.2 | v36.2,9.19 v30.8,9.19 v28.26,9.19 14.29,9.19 14.29,9.82 | 14.29,31.73 14.29,32.05 QG101.7 25.08,32.05 27.3,29.82 OK101.2 | OK201.5 v53.98,81.9
  Bottom 1.016: 79.69,68.24 C202.2
  Bottom 1.27: 17.78,86.66 15.24,86.66 14.29,85.7 v14.29,74.59 v14.29,64.75 v14.29,51.41 v14.29,50.14 v14.29,48.88 14.29,38.4 | 17.78,86.66 24.77,86.66 | 24.77,86.66 36.2,86.66 IC102.1 46.04,86.66 | 46.04,86.66 C104.- v52.07,83.8 v53.02,82.85 v53.98,81.9 | C103.- 49.09,89.7 46.04,86.66 | 24.77,86.66 V101.GND | 14.29,38.4 14.29,31.73 v14.29,31.41 v14.29,29.95 v14.29,28.55 14.29,20.93 | 14.29,20.93 14.29,9.82 14.29,9.51 | 14.29,9.51 14.29,9.19 14.29,3.47 v13.02,2.2 | v14.12,38.56 14.29,38.4 | v13.97,20.62 14.29,20.93 | 14.29,9.51 13.84,9.95 X101.4 X101.5 | CON101.2 7.5,94.79 8.89,96.18 13.34,96.18 17.46,92.06 17.46,86.98 17.78,86.66 | IC201.GND 79.69,61.26 | 79.69,61.26 C202.2 | v84.45,68.24 v83.19,68.24 v81.92,68.24 79.69,68.24 | 79.69,61.26 80.33,60.62 C201.2
  pour Bottom: 37.15,87.29 37.15,79.04 20,79.04 20,87.29
GNDI
  Bottom 1.016: 106.05,30.14 JP302.31
  Bottom 1.27: JP301.2 JP301.4 JP301.6 JP301.8 JP301.10 JP301.12 JP301.14 JP301.16 JP301.18 JP301.20 JP301.22 JP301.24 JP301.26 JP301.28 JP301.30 JP301.32 114.46,28.71 107.47,28.71 106.05,30.14 | JP302.1 JP302.3 JP302.5 JP302.7 JP302.9 JP302.11 JP302.13 JP302.15 JP302.17 JP302.19 JP302.21 JP302.23 JP302.25 JP302.27 JP302.29 JP302.31 106.05,29.51 107.31,28.24 107.31,23.48 106.2,22.36 SV301.2 SV301.4 SV301.6 SV301.8 SV301.10 SV301.12 SV301.14 SV301.16
GO
  Top 0.406: SV301.7 115.09,4.58 115.09,8.08 113.35,9.82 113.35,16.65 111.76,18.24 111.76,44.27 110.01,46.02 JP302.20
  Bottom 1.016: JP302.20 JP301.19
GO-I
  Bottom 0.61: IC101.28 54.45,46.33 56.04,44.75 68.58,44.75 69.85,46.02 71.91,46.02 T202.3
GO-O
  Bottom 0.61: IC101.29 R212.1
INIT
  Bottom 1.016: JP302.12 JP301.11
LED-G
  Top 0.406: R104.1 30.8,74.28 IC101.2
LED-R
  Top 0.406: R103.1 30.8,70.47 32.07,69.2 IC101.4
MISO  (via drill 0.5)
  Top 0.406: IC104.15 v48.9,9.19 48.9,10.14 47.62,11.41 47.62,13.95 45.72,15.86 v45.72,61.57 | IC103.2 66.04,19.66 67.31,18.39 v67.31,13.95
  Bottom 0.406: v45.72,61.57 IC101.7 | SV101.1 70.8,12.68 69.53,13.95 v67.31,13.95 63.18,13.95 58.42,9.19 v48.9,9.19
MOSI  (via drill 0.5)
  Top 0.406: IC104.14 v46.35,7.28 46.35,10.14 45.09,11.41 45.09,14.27 44.77,14.59 v44.77,64.12 | IC103.5 60.96,9.82 61.91,8.87 66.99,8.87 SV101.4
  Bottom 0.406: v44.77,64.12 IC101.6 | SV101.4 66.99,8.87 63.82,8.87 62.23,7.28 v46.35,7.28
N$1
  Bottom 0.406: IC105.1 30.8,13.32 34.29,16.81 55.56,16.81 56.52,15.86 IC104.1
N$2
  Bottom 0.406: IC105.4 23.18,11.09 23.81,10.46 53.34,10.46 53.98,11.09 IC104.2
N$3
  Bottom 0.61: R206.1 68.58,40.3 69.69,41.41 T201.2
N$4
  Bottom 0.61: R205.2 68.42,43.16 70.33,45.06 73.5,45.06 74.61,43.95 77.63,43.95 78.42,43.16 Q201.2
N$5
  Top 0.406: R108.1 20.64,28.24 21.27,28.87 24.77,28.87 25.4,28.24 25.4,25.06 27.3,23.16 OK101.3
N$7
  Bottom 0.61: R211.1 68.42,46.02 70.17,47.76 T202.2
N$9
  Top 0.406: R103.2 11.11,70.47 6.67,74.91 D101.AR
N$11  (via drill 0.5)
  Top 0.61: v10.48,25.06 20.32,25.06 22.54,27.29 R109.2
  Bottom 0.61: OK101.1 29.84,24.43 28.57,23.16 27.3,23.16 23.81,26.65 R109.2 | X101.3 3.11,8.93 1.91,10.14 1.91,19.35 3.17,20.62 9.84,20.62 10.48,21.25 v10.48,25.06
N$12
  Bottom 0.61: R212.2 67.94,49.03 70.8,51.89 76.36,51.89 78.42,49.83 Q203.2
N$13
  Top 0.406: R104.2 17.46,73.32 14.29,76.5 10.79,76.5 7.3,79.99 D101.AG
N$43
  Bottom 0.61: OK201.3 59.05,91.1 59.69,90.47 79.38,90.47 | 79.38,90.47 D202.A R207.1 | 79.38,90.47 D201.A
N$53
  Bottom 0.61: Q204.1 70.48,79.67 Q202.2 60.64,74.91 59.37,73.64 R209.2
N$54
  Top 0.61: Q204.2 70.48,78.09 Q202.3
  Bottom 0.61: Q202.3 71.75,73.01 71.12,72.37 63.18,72.37 62.23,71.42 R208.1
N$56
  Bottom 0.61: Q204.3 69.22,83.8 69.69,84.28 72.39,84.28 72.87,83.8 73.03,83.8 73.18,83.64 73.18,72.69 70.33,69.83 R210.1
N$57
  Top 0.61: R210.2 62.87,79.99 | OK201.2 61.59,91.1 62.87,89.83 62.87,79.99 | 62.87,79.99 R208.2
NC
  Bottom 1.016: JP302.16 JP301.15
PLUGGED  (via drill 0.5)
  Top 0.406: v10.48,73.01 15.24,73.01 16.19,72.05 30.8,72.05 31.75,73.01 36.83,73.01 v38.1,74.28
  Bottom 0.406: CON101.3 10.65,73.18 v10.48,73.01 | v38.1,74.28 IC101.39
ROT  (via drill 0.5)
  Top 0.61: D201.C 69.22,91.74 67.31,89.83 v67.31,86.02 67.31,84.91 67.94,84.28 72.55,84.28 72.87,83.96 81.12,83.96 82.55,85.39 X201.2
  Bottom 0.61: 67.31,76.81 60.96,76.81 59.37,78.4 R209.1 | Q202.1 67.31,76.81 | 67.31,76.81 v67.31,86.02
SCK  (via drill 0.5)
  Top 0.406: IC104.13 v43.81,8.24 43.81,10.14 42.55,11.41 42.55,13.95 43.81,15.22 v43.81,59.03 | IC103.6 v63.5,12.36
  Bottom 0.406: v43.81,59.03 IC101.8 | SV101.3 68.26,11.73 67.31,12.68 63.82,12.68 v63.5,12.36 59.37,8.24 v43.81,8.24
SCL
  Top 0.406: SV301.3 110.01,4.58 110.01,22.21 110.17,22.36 110.17,34.75 109.06,35.86 JP302.28
  Bottom 1.016: JP302.28 JP301.27
SDA
  Top 0.406: SV301.1 107.47,4.58 107.47,21.09 109.38,23 109.38,29.98 JP302.32
  Bottom 1.016: JP302.32 JP301.31
SPG  (via drill 0.5)
  Top 0.406: v46.67,67.92 v46.67,76.81
  Bottom 0.406: v46.67,67.92 30.16,67.92 R106.2 R107.1 | v46.67,76.81 IC101.40
STOP
  Top 0.406: SV301.5 112.55,4.58 112.55,16.33 110.97,17.92 110.97,40.14 110.17,40.94 JP302.24
  Bottom 1.016: JP302.24 JP301.23
STOP-I
  Bottom 0.61: IC101.25 56.67,38.71 56.83,38.87 71.12,38.87 T201.3
STOP-O
  Bottom 0.61: IC101.26 53.82,41.25 55.72,43.16 R205.1
TRACK  (via drill 0.5)
  Top 0.406: v40.01,78.09 40.01,43.79 40.01,39.83 38.89,38.71 IC101.16
  Bottom 0.406: v40.01,78.09 54.61,78.09 R213.2 59.05,82.53 OK201.6
V+  (via drill 0.5)
  Top 0.813: C105.1 31.75,84.75 29.84,86.66
  Top 1.27: V101.IN 29.84,86.34 29.84,86.66 D102.C 29.84,89.52 30.48,90.15 42.55,90.15 43.18,90.79 43.18,93.64 43.81,94.28 46.67,94.28 47.31,93.64 47.31,85.07 46.35,84.12 C104.+ 46.35,82.85 47.94,81.26 50.16,81.26 51.75,79.67 v51.75,76.81 v51.75,75.55 v51.75,74.28
  Bottom 1.27: C201.1 79.38,51.89 77.15,54.11 77.15,55.22 | IC201.IN 77.15,57.29 77.15,55.22 | 77.15,55.22 57.47,55.22 53.98,58.72 53.98,71.1 51.75,73.32 v51.75,74.28 v51.75,75.55 v51.75,76.81
V-NETZTEIL
  Top 1.27: D103.A 23.18,93.33 21.27,91.42 14.6,91.42 CON101.1

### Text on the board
Bottom: mbc89.brd | bottom | MBCAN-Projekt | 01.03.2022 | (c) Dr.-Ing. Th. Wiesner | (c) Dr.-Ing. Th. Wiesner | mbc89.brd | bottom
tNames: HW: 22.03.01 | I2C-Bus / Märklin Digital 1. Generation | 0 | B | +18V | DC | STATUS | sonstige MM-Zentralen | (c) Dr.-Ing. Th. Wiesner | MBCAN-Projekt | I2C-Bus Märklin Digital 1. Generation | IN | *) Bei Bedarf | BL | FL | (c) Dr.-Ing. Th. Wiesner | OUT | MBCAN-Projekt | 6021 | 6040/6043 | mbc-89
